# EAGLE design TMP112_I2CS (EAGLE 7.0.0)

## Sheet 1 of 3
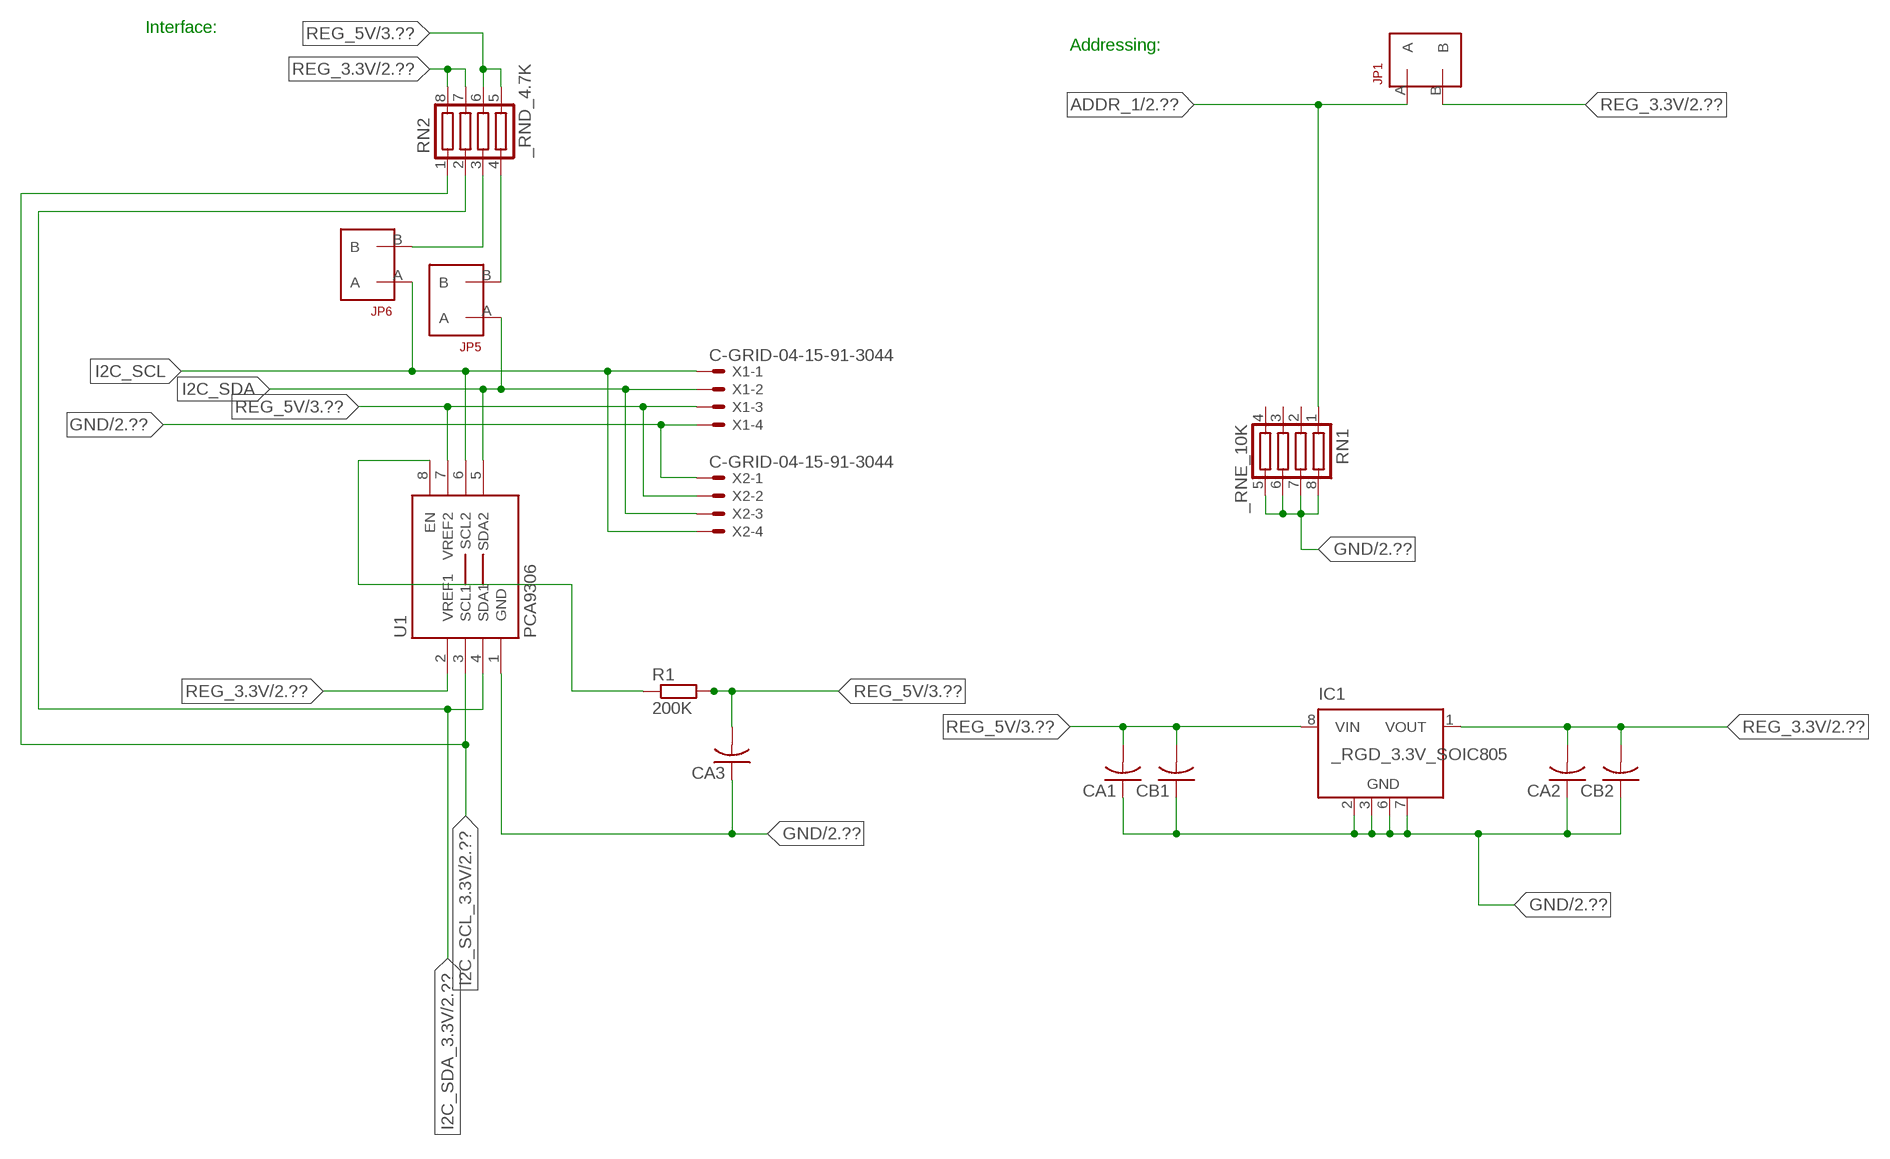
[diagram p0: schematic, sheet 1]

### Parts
CA1  CC1206KRX7R9BB104  [.1UF]
CA2  CC1206KRX7R9BB104  [.1UF]
CA3  CC1206KRX7R9BB104  [.1UF]
CB1  TMK316F106ZL-TC1206K  [TMK316F106ZL-T]
CB2  TMK316F106ZL-TC1206K  [TMK316F106ZL-T]
IC1  _RGD_3.3V_SOIC805  [_RGC_3.3V_SOIC8]
JP1  JUMPER_1X2_2MM  [JUMPER_1X2_2MM]
JP5  JUMPER_1X2_2MM  [JUMPER_1X2_2MM]
JP6  JUMPER_1X2_2MM  [JUMPER_1X2_2MM]
R1  200K  RESISTOR_SMT-0603  [R603]
RN1  _RNE_10K  [RNE]
RN2  _RND_4.7K  [RND]
U1  PCA9306  PCA9306_NCD  [PSOP-8]
X1  C-GRID-04-15-91-3044  [15-91-04]
X2  C-GRID-04-15-91-3044  [15-91-04]

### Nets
ADDR_1: JP1.A RN1.1 ; also sheet 2
GND: CA1.1 CA2.1 CA3.1 CB1.1 CB2.1 IC1.2(GND) IC1.3(GND) IC1.6(GND) IC1.7(GND) RN1.5 RN1.6 RN1.7 RN1.8 U1.1(GND) X1.4 X2.1 ; also sheet 2,3
I2C_SCL: JP6.A U1.6(SCL2) X1.1 X2.4
I2C_SCL_3.3V: RN2.1 U1.3(SCL1) ; also sheet 2
I2C_SDA: JP5.A U1.5(SDA2) X1.2 X2.3
I2C_SDA_3.3V: RN2.2 U1.4(SDA1) ; also sheet 2
N$1: JP6.B RN2.3
N$2: JP5.B RN2.4
N$23: R1.1 U1.8(EN)
REG_3.3V: CA2.2 CB2.2 IC1.1(VOUT) JP1.B RN2.7 RN2.8 U1.2(VREF1) ; also sheet 2
REG_5V: CA1.2 CA3.2 CB1.2 IC1.8(VIN) R1.2 RN2.5 RN2.6 U1.7(VREF2) X1.3 X2.2 ; also sheet 3
Unconnected: IC1.4(NC) IC1.5(NC) RN1.2 RN1.3 RN1.4

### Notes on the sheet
- Interface:
- Addressing:

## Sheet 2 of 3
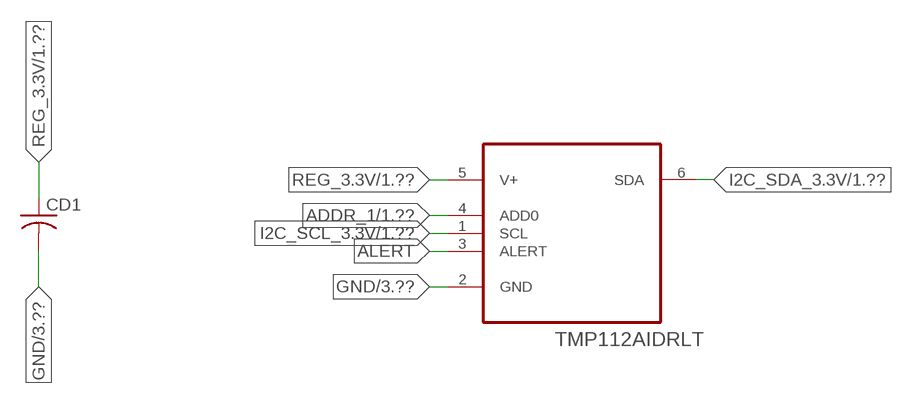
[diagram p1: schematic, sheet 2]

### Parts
CD1  CC1206KRX7R9BB103C1206K  [CC1206KRX7R9BB103]
IC2  TMP112AIDRLT  [SOT50P120X60-6N]

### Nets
ADDR_1: IC2.4(ADD0) ; also sheet 1
ALERT: IC2.3(ALERT)
GND: CD1.2 IC2.2(GND) ; also sheet 1,3
I2C_SCL_3.3V: IC2.1(SCL) ; also sheet 1
I2C_SDA_3.3V: IC2.6(SDA) ; also sheet 1
REG_3.3V: CD1.1 IC2.5(V+) ; also sheet 1

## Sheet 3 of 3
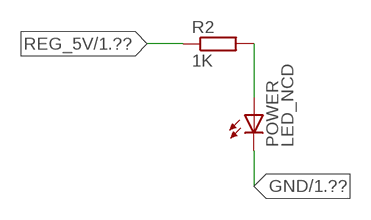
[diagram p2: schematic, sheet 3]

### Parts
POWER  LED_NCD  [CHIPLED_0603]
R2  1K  RESISTOR_SMT-0402  [R402]

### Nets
GND: POWER.C ; also sheet 1,2
N$4: POWER.A R2.2
REG_5V: R2.1 ; also sheet 1

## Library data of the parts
CA1-CA3 = NCD_ULTIMATE_LIBRARY:CC1206KRX7R9BB104: Capacitor CA .1uF 50V SMT C1206K CC1206KRX7R9BB104
CB1 CB2 = NCD_ULTIMATE_LIBRARY:TMK316F106ZL-T: Capacitor CB 10uF SMT 1206 TMK316F106ZL-T
CD1 = NCD_ULTIMATE_LIBRARY:CC1206KRX7R9BB103: Capacitor CD .01uF SMT CC1206KRX7R9BB103 1206
IC1 = NCD_ULTIMATE_LIBRARY:_RGD_3.3V_SOIC8: Regulator Linear 3.3V Chip Positive VOLTAGE REGULATOR Digikey 497-1199-2-ND/L78L33ACD13TR
IC2 = Texas Instruments_By_element14_Batch_1:TMP112AIDRLT: Digital Temperature Sensor; MPN: TMP112AIDRLT; OC_FARNELL: 1735574; OC_NEWARK: 14R8030; PACKAGE: SOT563-6; SUPPLIER: TEXAS INSTRUMENTS
JP1 JP5 JP6 = NCD_ULTIMATE_CONNECTORS:JUMPER_1X2_2MM
POWER = NCD_ULTIMATE_LIBRARY:LED_NCD: LED Digikey 754-1132-2-ND/APT2012SRCPRV
R1 R2 = NCD_ULTIMATE_LIBRARY:RESISTOR_SMT: NCD Resistor
RN1 = NCD_ULTIMATE_LIBRARY:_RNE_10K: Resistor Array RNE SMT 10K x 4 Single Resistor Source: http://www.ctscorp.com/components/Datasheets/CTSChipArrayDs.pdf Digikey 742C083103JPTR-ND/742C083103JP; OC_FARNELL: unknown; OC_NEWARK: unknown
RN2 = NCD_ULTIMATE_LIBRARY:_RND_4.7K: Resistor Array RND SMT 4.7K x 4 Single Resistor Source: http://www.ctscorp.com/components/Datasheets/CTSChipArrayDs.pdf Digikey 742C083472JPTR-ND/742C083472JP; OC_FARNELL: unknown; OC_NEWARK: unknown
U1 = NCD_ULTIMATE_LIBRARY:PCA9306_NCD: NCD Bidirectional I2C level shifter. NOT compatible with all available part number pinout schemes- DOUBLE CHECK!!!; PROD_ID: IC-10023
X1 X2 = NCD_ULTIMATE_CONNECTORS:C-GRID-04: CONNECTOR 4-Pos I2C wire to board 2.54 mm (0.100") pitch header Digikey WM1342-ND/0015912045; OC_FARNELL: unknown; OC_NEWARK: unknown

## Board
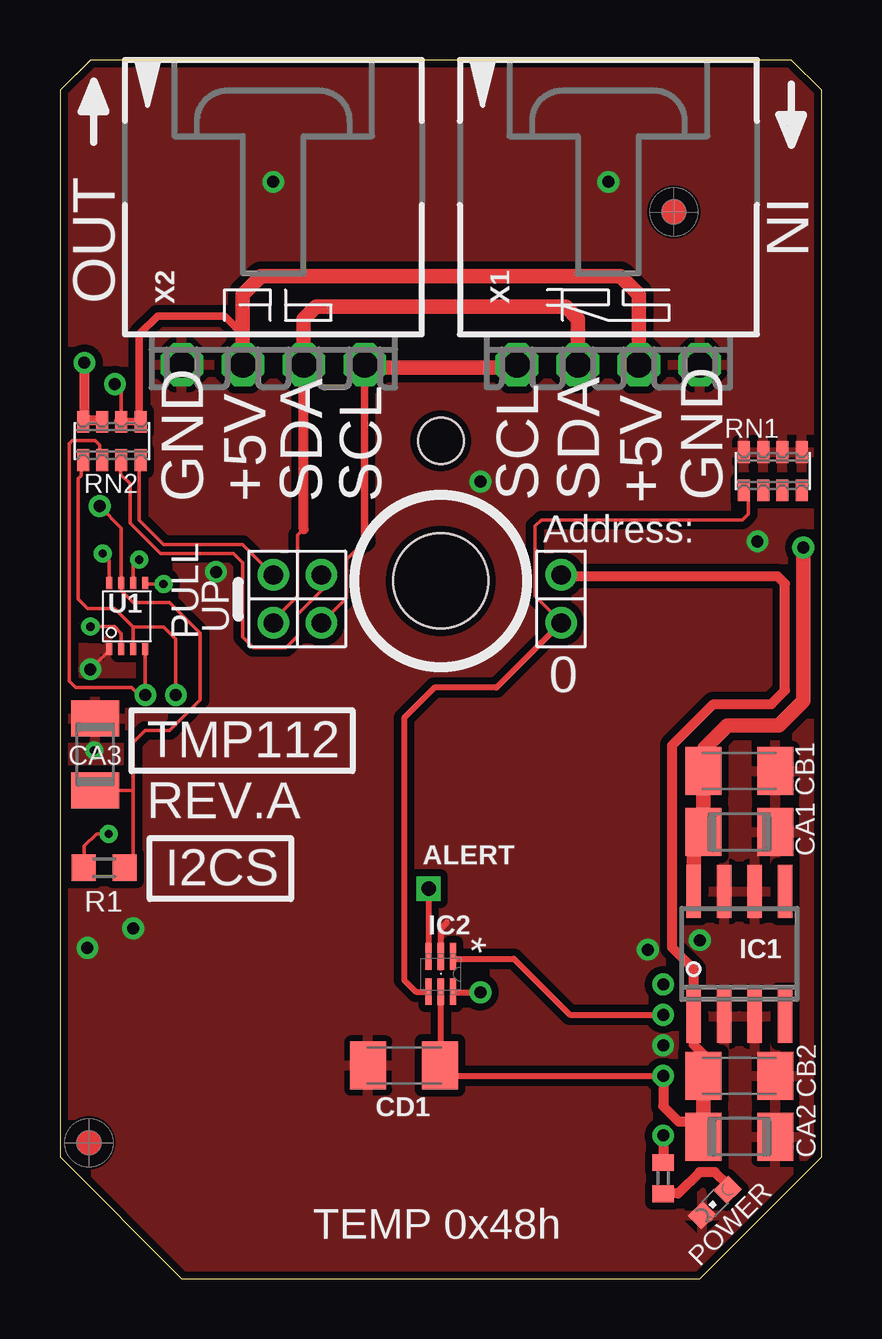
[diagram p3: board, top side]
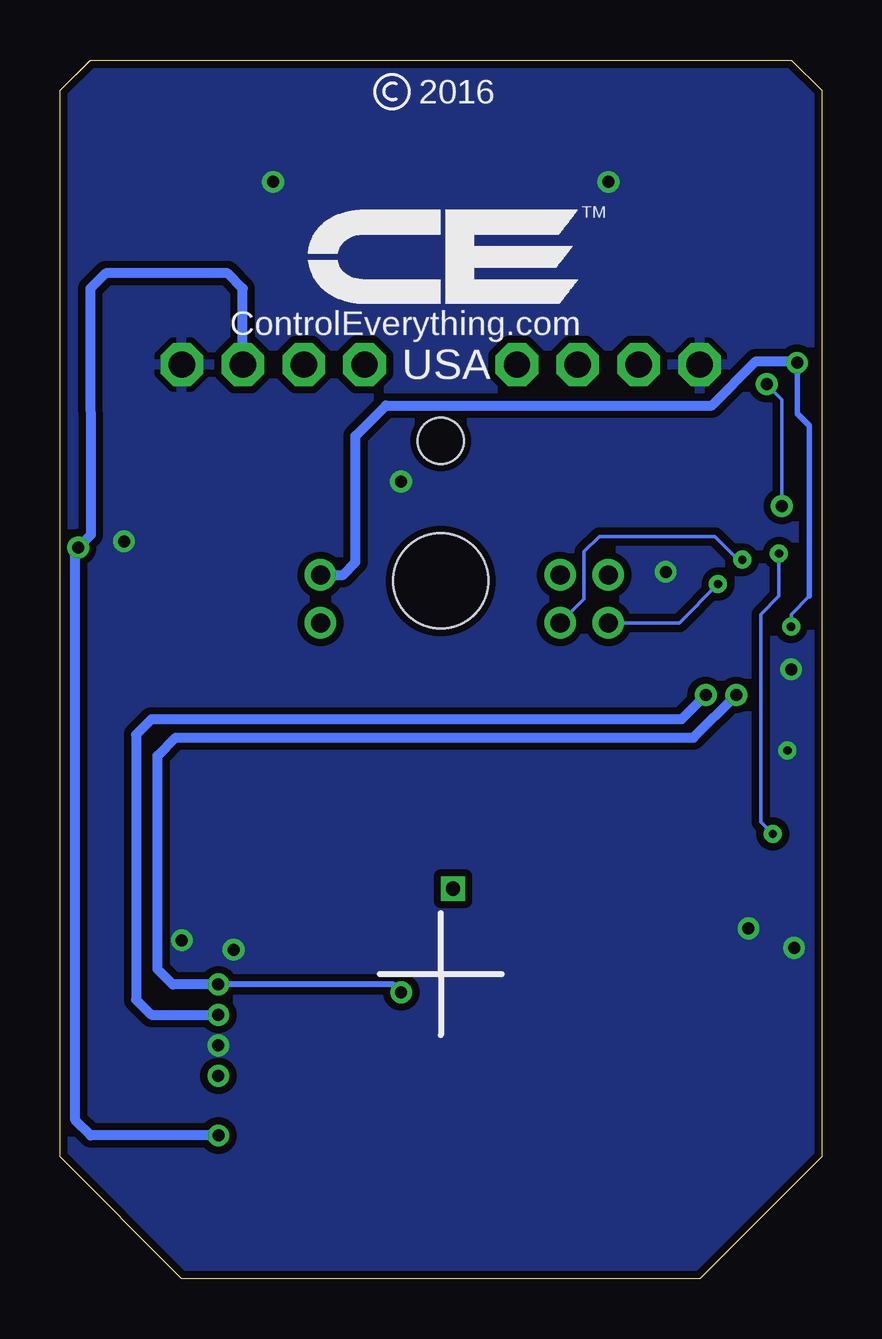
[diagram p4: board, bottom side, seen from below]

Size 31.75 x 50.8 mm. Coordinates in mm from the lower left corner, seen from the top.
Outline: 48 segments
Copper layers (1*16): Top 0.035mm / dielectric 1.5mm / Bottom 0.035mm
Design rules "default": minimum track width 5mil, minimum drill 24mil, track to track 5mil, track to pad 5mil, pad to pad 5mil, via to via 5mil, smd to smd 5mil, copper to edge 10mil, drill to drill 8mil, minimum pad ring 10mil, minimum via ring 8mil, stop-mask expansion 2mil, vias tented up to drill 0mil, thermal gap 10mil
Holes 3.96 mm at 15.88,29.08
Holes 1.91 mm at 15.88,34.93

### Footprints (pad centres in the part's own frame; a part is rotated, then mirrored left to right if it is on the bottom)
.1UF = smd 1.5 x 2: 1 -1.5,0; 2 1.5,0
TMK316F106ZL-T = smd 1.5 x 2: 1 -1.5,0; 2 1.5,0
CC1206KRX7R9BB103 = smd 1.5 x 2: 1 -1.5,0; 2 1.5,0
_RGC_3.3V_SOIC8 = smd 0.6 x 2.2: 1 -1.905,-2.6; 2 -0.635,-2.6; 3 0.635,-2.6; 4 1.905,-2.6; 5 1.905,2.6; 6 0.635,2.6; 7 -0.635,2.6; 8 -1.905,2.6
SOT50P120X60-6N = smd 1.118 x 0.254: 1 -0.737,0.508; 2 -0.737,0; 3 -0.737,-0.508; 4 0.737,-0.508; 5 0.737,0; 6 0.737,0.508
JUMPER_1X2_2MM = drill 0.8: A 0,2; B 0,0
CHIPLED_0603 = smd 0.8 x 0.876: A 0,-0.75; C 0,0.75
R603 = smd 1 x 1.1: 1 -0.85,0; 2 0.85,0
R402 = smd 0.7 x 0.9: 1 -0.65,0; 2 0.65,0
RNE = smd 0.5 x 0.9: 1 -1.2,-0.8; 2 -0.4,-0.8; 3 0.4,-0.8; 4 1.2,-0.8; 5 1.2,0.8; 6 0.4,0.8; 7 -0.4,0.8; 8 -1.2,0.8
RND = smd 0.5 x 0.9: 1 -1.2,-0.8; 2 -0.4,-0.8; 3 0.4,-0.8; 4 1.2,-0.8; 5 1.2,0.8; 6 0.4,0.8; 7 -0.4,0.8; 8 -1.2,0.8
PSOP-8 = smd 0.25 x 0.5: 1 -0.73,-1.37; 2 -0.23,-1.37; 3 0.27,-1.37; 4 0.77,-1.37; 5 0.77,1.38; 6 0.27,1.38; 7 -0.23,1.38; 8 -0.73,1.38
15-91-04 = drill 1.1 pad 1.778 octagon: 1 -3.81,-7.62; 2 -1.27,-7.62; 3 1.27,-7.62; 4 3.81,-7.62

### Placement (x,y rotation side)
CA1  28.32,18.62 180 top
CA2  28.32,5.92 180 top
CA3  1.46,21.86 270 top
CB1  28.32,21.16 180 top
CB2  28.32,8.46 180 top
CD1  14.35,8.89 180 top
IC1  28.32,13.54 0 top
IC2  15.88,12.7 270 top
JP1  20.89,29.34 180 top
JP5  8.89,29.34 180 top
JP6  10.9,29.34 180 top
POWER  27.3,3.18 135 top
R1  1.84,17.13 0 top
R2  25.15,4.19 270 top
RN1  29.72,33.66 0 top
RN2  2.16,34.93 0 top
U1  2.79,27.61 0 top
U$5  [VISION_REF10]  1.21,5.66 90 top
U$28  [VISION_REF10]  25.59,44.46 90 top
X1  22.86,45.72 0 top
X2  8.89,45.72 0 top

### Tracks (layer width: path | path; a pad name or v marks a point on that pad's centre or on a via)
ADDR_1
  Top 0.152: JP1.A 20.89,27.37 19.81,28.45 19.81,31.37 20.07,31.62 28.45,31.62 28.7,31.88 28.7,32.78 RN1.1
  Top 0.254: JP1.A 18.2,24.64 15.62,24.64 14.35,23.37 14.35,12.45 14.83,11.96 IC2.4
ALERT  (via drill 0.6)
  Top 0.254: v15.37,16.26 IC2.3
GND  (via drill 0.35, 0.5)
  Top 0.152: CA3.1 1.52,23.42 1.52,23.62 | v1.27,25.4 2.06,26.19 U1.1
  Top 0.254: IC2.2 15.88,14.61 16.13,14.86
  other vias: 8.89,45.72 22.86,45.72 25.15,9.73 17.53,33.22 26.67,14.11 1.15,13.79 6.5,29.46 3.05,14.61 24.51,13.72 1.42,22.02 29.08,30.73
  pour Bottom (isolate 0.305): -0.64,5.08 -0.64,49.53 1.27,51.44 30.48,51.44 32.38,49.53 32.38,5.08 26.67,-0.63 5.08,-0.63
  pour Top (isolate 0.305): 4.45,-1.27 -1.27,4.45 -1.27,50.17 0.64,52.07 31.11,52.07 33.02,50.17 33.02,4.45 27.3,-1.27
I2C_SCL  (via drill 0.35)
  Top 0.152: 12.7,30.73 11.94,29.97 11.94,28.38 JP6.A | v3.3,29.97 3.06,29.73 U1.6
  Top 0.305: 12.7,30.73 X2.4
  Top 0.406: X2.4 12.7,37.97 | 19.05,37.97 X1.1
  Top 0.61: 12.7,37.97 19.05,37.97
  Bottom 0.152: JP6.A 9.91,28.33 9.91,30.3 9.27,30.94 4.45,30.94 3.48,29.97 v3.3,29.97
I2C_SCL_3.3V  (via drill 0.5)
  Top 0.152: RN2.1 0.89,34.07 0.89,33.48 0.77,33.35 0.77,28.33 1.16,27.94 2.29,27.94 3.06,27.17 | 3.06,27.17 U1.3 | v4.83,24.33 v4.83,24.34 4.83,26.67 4.33,27.17 3.06,27.17
  Top 0.254: IC2.1 16.48,13.34 18.92,13.34 21.26,11 v25.15,11
  Bottom 0.406: v4.83,24.33 5.84,23.32 27.94,23.32 28.58,22.68 28.58,11.63 27.94,11 v25.15,11
I2C_SDA  (via drill 0.35)
  Top 0.152: JP5.A 8.89,27.44 9.91,28.45 9.91,30.99 10.16,31.24 | U1.5 3.6,28.96 v4.32,28.96
  Top 0.406: 10.16,31.24 X2.3
  Top 0.61: X2.3 10.16,40.01 10.67,40.51 21.09,40.51 21.59,40.01 X1.2
  Bottom 0.152: v4.32,28.96 5.94,27.34 JP5.A
I2C_SDA_3.3V  (via drill 0.5)
  Top 0.152: RN2.2 1.65,34.14 1.65,34.75 1.46,34.94 0.51,34.94 0.38,34.81 0.38,26.37 0.38,26.36 0.38,24.92 0.66,24.64 3,24.64 3.3,24.33 v3.56,24.33 U1.4
  Top 0.254: IC2.6 16.41,11.94 v17.53,11.94
  Bottom 0.254: v17.53,11.94 17.86,12.27 v25.15,12.27
  Bottom 0.406: v25.15,12.27 27.05,12.27 27.69,12.9 27.69,21.79 26.93,22.56 5.34,22.56 v3.56,24.33
N$1
  Top 0.152: JP6.B 10.92,29.31 10.92,28.7 9.91,27.69 9.91,26.8 9.42,26.31 8.06,26.31 7.62,26.75 7.62,29.84 7.24,30.23 4.19,30.23 2.92,31.5 2.92,33.15 2.54,33.53 2.54,34.1 RN2.3
  Top 0.305: 2.54,34.02 RN2.3
N$2
  Top 0.152: JP5.B 7.62,30.61 4.32,30.61 3.3,31.62 3.3,34.07 RN2.4
  Top 0.305: 3.37,33.88 RN2.4
N$4
  Top 0.406: POWER.A 27.84,3.92 27.3,4.45 26.67,4.45 25.78,3.56 25.16,3.56 R2.2
N$23  (via drill 0.35)
  Top 0.152: R1.1 1.02,17.16 1.02,18.03 1.52,18.54 v2.03,18.54 | v1.78,30.23 2.06,29.94 U1.8
  Bottom 0.152: v2.03,18.54 2.54,19.05 2.54,27.69 1.78,28.45 v1.78,30.23
REG_3.3V  (via drill 0.35, 0.5)
  Top 0.152: v1.27,27.18 2.29,27.18 2.56,26.9 U1.2
  Top 0.254: IC2.5 15.88,8.91 CD1.1 16.28,8.46 v25.15,8.46
  Top 0.406: CB2.2 26.82,9.35 26.42,9.75 26.42,10.36 | v25.15,8.46 25.15,7.19 25.78,6.55 26.82,6.55 | IC1.1 26.42,12.9 25.53,13.79 25.53,22.24 27.24,23.95 29.66,23.95 30.23,24.52 30.23,28.97 29.91,29.29 20.95,29.29 JP1.B | 26.52,5.62 CA2.2 | v1.02,38.18 1.02,35.78 | 1.02,35.78 RN2.8 | 1.02,35.78 1.71,35.78 RN2.7
  Top 0.61: CB2.2 26.82,6.55 CA2.2 | 26.42,10.36 IC1.1
  Bottom 0.152: 0.51,28.45 1.27,27.69 v1.27,27.18
  Bottom 0.229: 0.51,28.45 0.51,35.56 1.02,36.07 v1.02,38.18
  Bottom 0.406: v1.02,38.18 1.08,38.24 2.73,38.24 4.58,36.4 18.16,36.4 19.43,35.13 19.43,29.87 19.94,29.34 JP1.B
REG_5V  (via drill 0.5)
  Top 0.152: RN2.6 2.56,37.01 v2.29,37.29 | R1.2 3.05,17.49 3.05,20.36 | 3.05,20.36 3.05,22.35 3.56,22.86 4.57,22.86 5.84,24.13 5.84,26.92 4.57,28.19 3.05,28.19 2.56,28.68 U1.7 2.56,31.3 v1.65,32.21 | CA3.2 3.05,20.36
  Top 0.305: 7.62,39.37 7.5,39.37 | 2.42,35.74 RN2.6 RN2.5 3.31,35.8 3.31,39.37 4.07,40.13 6.86,40.13 7.62,39.37 | X2.2 7.62,39.37
  Top 0.406: v25.15,5.97 R2.1
  Top 0.61: X1.3 24.13,41.02 23.37,41.78 8.38,41.78 7.62,41.02 X2.2 | IC1.8 26.42,18.21 CA1.2 CB1.2 26.86,21.2 26.86,22.11 27.82,23.06 29.98,23.06 30.99,24.08 v30.99,30.48
  Bottom 0.152: v1.65,32.21 1.65,36.65 v2.29,37.29
  Bottom 0.406: X1.3 24.13,41.28 24.77,41.91 29.84,41.91 30.48,41.27 30.47,31 v30.99,30.48 31.11,30.36 31.11,6.6 30.48,5.97 v25.15,5.97

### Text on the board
tNames: IN | OUT | GND | +5V | SDA | SCL | SCL | SDA | +5V | GND | Address: | PULL | UP | 0 | TMP112 | REV.A | ALERT | I2CS | TEMP 0x48h
bNames: 2016 | TM | ControlEverything.com | USA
